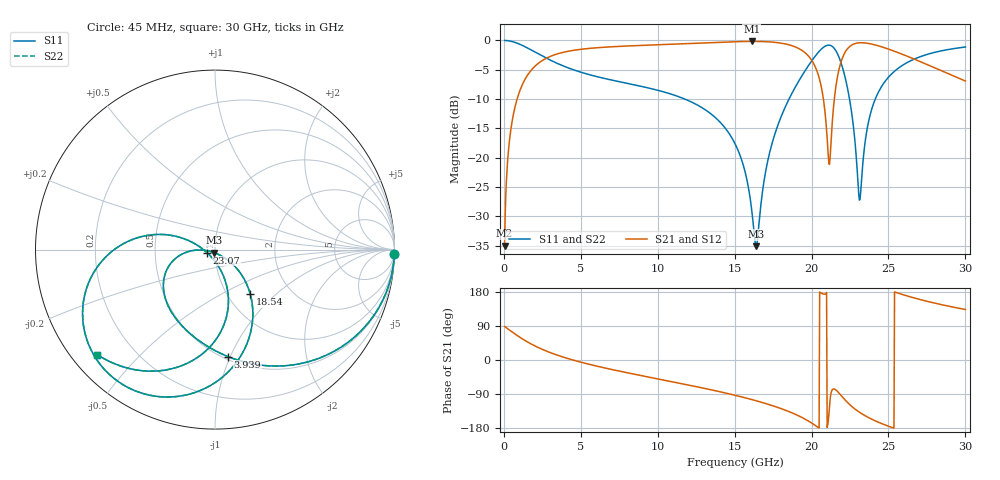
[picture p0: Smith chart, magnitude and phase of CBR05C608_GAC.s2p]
! S-parameter model data by Modelithics Inc.  support@modelithics.com 813-866-6335  Tampa FL USA
! S-Parameter data specifications:
! Substrate: 20-mil Rogers 4350B, substrate thickness, H=0.508mm, Dielectric constant, Er=3.75
! PCB Mounting Pad Footprint: Pad width, PadW=1.79mm , Pad length, PadL=0.95mm , Pad gap, PadG (edge-to-edge)=0.69mm , Reference planes=2.59mm apart
#  GHz  S  MA  R 50
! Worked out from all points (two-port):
!   801 points, 45 MHz to 30 GHz, reference 50 ohm
!   highest |S21| = -0.16 dB at 16.11 GHz (marker M1); lowest = -35.0 dB at 45 MHz (marker M2)
!   |S21| within 3 dB of the highest: 2.666 GHz to 19.95 GHz (17.28 GHz wide, 153 % of centre); 21.98 GHz to 26.65 GHz (4.673 GHz wide, 19.2 % of centre)
!   lowest |S11| = -35.1 dB at 16.41 GHz (marker M3), VSWR 1.04, Z = 49.5 - j1.67 ohm
!   |S11| at or under -10 dB: 11.76 GHz to 18.53 GHz (6.777 GHz wide, 44.7 % of centre); 22.47 GHz to 24.14 GHz (1.675 GHz wide, 7.19 % of centre)
!   |S22| runs from -35.1 to 0.0 dB; largest |S21 - S12| = 0
!   S11 on the Smith chart (normalised r, x): 45 MHz: 1, -84; 3.939 GHz: 0.53, -0.98; 18.54 GHz: 1.27, -0.71; 23.07 GHz: 0.91, -0.03; 30 GHz: 0.07, -0.38
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0.045  0.9998 -1.4  0.01775 88.5  0.01775 88.5  0.9998 -1.4
0.381994  0.9886 -11.5  0.148 78.4  0.148 78.4  0.9886 -11.5
1.018538  0.9295 -29.5  0.367 60.4  0.367 60.4  0.9295 -29.5
2.14185  0.7801 -55.2  0.6234 34.6  0.6234 34.6  0.7801 -55.2
3.93915  0.6001 -83.2  0.7965 6.6  0.7965 6.6  0.6001 -83.2
5.062462  0.5328 -96.0  0.8421 -6.4  0.8421 -6.4  0.5328 -96.0
10.04248  0.3745 -139.2  0.9194 -50.2  0.9194 -50.2  0.3745 -139.2
15.0225  0.1316 -177.0  0.9762 -93.0  0.9762 -93.0  0.1316 -177.0
16.10837  0.03574 -166.6  0.9814 -104.3  0.9814 -104.3  0.03574 -166.6
16.40792  0.01757 -105.8  0.981 -107.6  0.981 -107.6  0.01757 -105.8
17.23168  0.1046 -39.0  0.9724 -117.6  0.9724 -117.6  0.1046 -39.0
18.54221  0.3178 -51.7  0.9172 -136.4  0.9172 -136.4  0.3178 -51.7
20.03996  0.6781 -83.1  0.667 -167.3  0.667 -167.3  0.6781 -83.1
20.63906  0.8442 -104.3  0.3986 176.4  0.3986 176.4  0.8442 -104.3
21.16327  0.9112 -130.2  0.08754 -124.3  0.08754 -124.3  0.9112 -130.2
21.87471  0.6687 -171.1  0.6293 -91.6  0.6293 -91.6  0.6687 -171.1
22.54869  0.2718 162.6  0.9022 -120.2  0.9022 -120.2  0.2718 162.6
23.07291  0.04762 -159.2  0.954 -136.8  0.954 -136.8  0.04762 -159.2
23.85922  0.2455 -73.1  0.9342 -155.2  0.9342 -155.2  0.2455 -73.1
25.01998  0.489 -88.4  0.8421 -175.1  0.8421 -175.1  0.489 -88.4
27.15427  0.7337 -113.4  0.6522 158.5  0.6522 158.5  0.7337 -113.4
30  0.8789 -138.2  0.4505 133.3  0.4505 133.3  0.8789 -138.2
